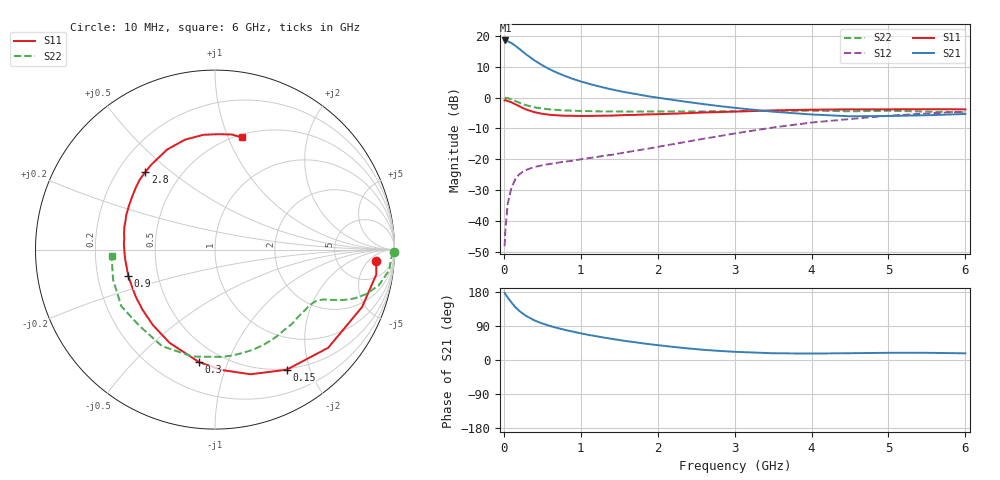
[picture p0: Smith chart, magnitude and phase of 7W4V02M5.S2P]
! Infineon Technologies  Discrete & RF Semiconductors
! BFS17W
! Si NPN RF Bipolar Junction Transistor in SOT323
! VCE = 4 V  IC = 2.5 mA
! Common Emitter S-Parameters:  August  1999
# GHz  S  MA  R  50
!  f  S11  S21  S12  S22
! GHz  MAG  ANG  MAG  ANG  MAG  ANG  MAG  ANG
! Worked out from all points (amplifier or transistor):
!   36 points, 10 MHz to 6 GHz, reference 50 ohm
!   highest |S21| = 18.5 dB at 20 MHz (marker M1)
!   |S21| within 3 dB of that: start of sweep to 214.7 MHz
!   unconditionally stable (mu >= 1): 765.1 MHz to 3.09 GHz; 4.112 GHz to end of sweep
!   at 250 MHz: K = 0.40, MSG = 19.4 dB, |S12| = -24.0 dB
!   at 1.4 GHz: K = 1.29, MAG = 7.4 dB, |S12| = -18.6 dB
!   at 6 GHz: K = 1.09, MAG = -2.2 dB, |S12| = -4.6 dB
!   S11 on the Smith chart (normalised r, x): 10 MHz: 13, -9; 150 MHz: 0.49, -1.65; 300 MHz: 0.38, -0.79; 900 MHz: 0.34, -0.13; 2.8 GHz: 0.31, +0.41; 6 GHz: 0.53, +1.12
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0.01  0.9005 -4.2  8.364 177.6  0.0039 83.3  0.9982 -0.9
0.02  0.9091 -8.8  8.41 174.0  0.0071 93.9  0.982 -2.7
0.05  0.8798 -21.3  8.168 164.9  0.0189 80.2  0.9783 -6.7
0.1  0.8348 -40.9  7.615 151.5  0.035 69.2  0.9338 -12.3
0.15  0.7793 -59.2  6.894 139.4  0.0475 60.3  0.8779 -16.4
0.2  0.7221 -74.1  6.169 129.7  0.0568 54.6  0.8256 -19.2
0.25  0.6722 -86.7  5.469 121.8  0.063 49.3  0.7797 -21.0
0.3  0.6333 -98.1  4.894 115.1  0.0679 47.0  0.7453 -22.2
0.4  0.5777 -116.0  3.984 104.4  0.075 43.6  0.6932 -23.8
0.5  0.5447 -129.4  3.331 96.4  0.0797 42.3  0.6623 -24.8
0.6  0.5247 -140.3  2.849 89.8  0.0839 42.5  0.6418 -26.1
0.7  0.5139 -149.1  2.499 84.2  0.0879 43.2  0.6278 -27.5
0.9  0.5048 -163.2  2 74.7  0.0947 45.8  0.6095 -31.0
1.1  0.5034 -174.2  1.679 66.3  0.104 49.3  0.602 -35.0
1.3  0.5083 176.7  1.45 59.2  0.1138 52.5  0.5952 -39.7
1.6  0.5209 165.6  1.206 49.7  0.1301 57.0  0.5919 -46.9
2.2  0.5471 147.8  0.914 34.6  0.1756 63.5  0.5955 -63.2
2.8  0.5807 132.0  0.727 24.0  0.2367 65.2  0.5976 -80.7
3.5  0.6182 115.5  0.589 17.8  0.327 61.8  0.6089 -101.8
4.5  0.6429 95.7  0.497 17.9  0.448 50.0  0.5982 -134.5
5.5  0.6479 81.7  0.516 19.0  0.5504 37.2  0.592 -163.5
6  0.6427 76.5  0.541 17.6  0.59 30.9  0.5778 -176.2
